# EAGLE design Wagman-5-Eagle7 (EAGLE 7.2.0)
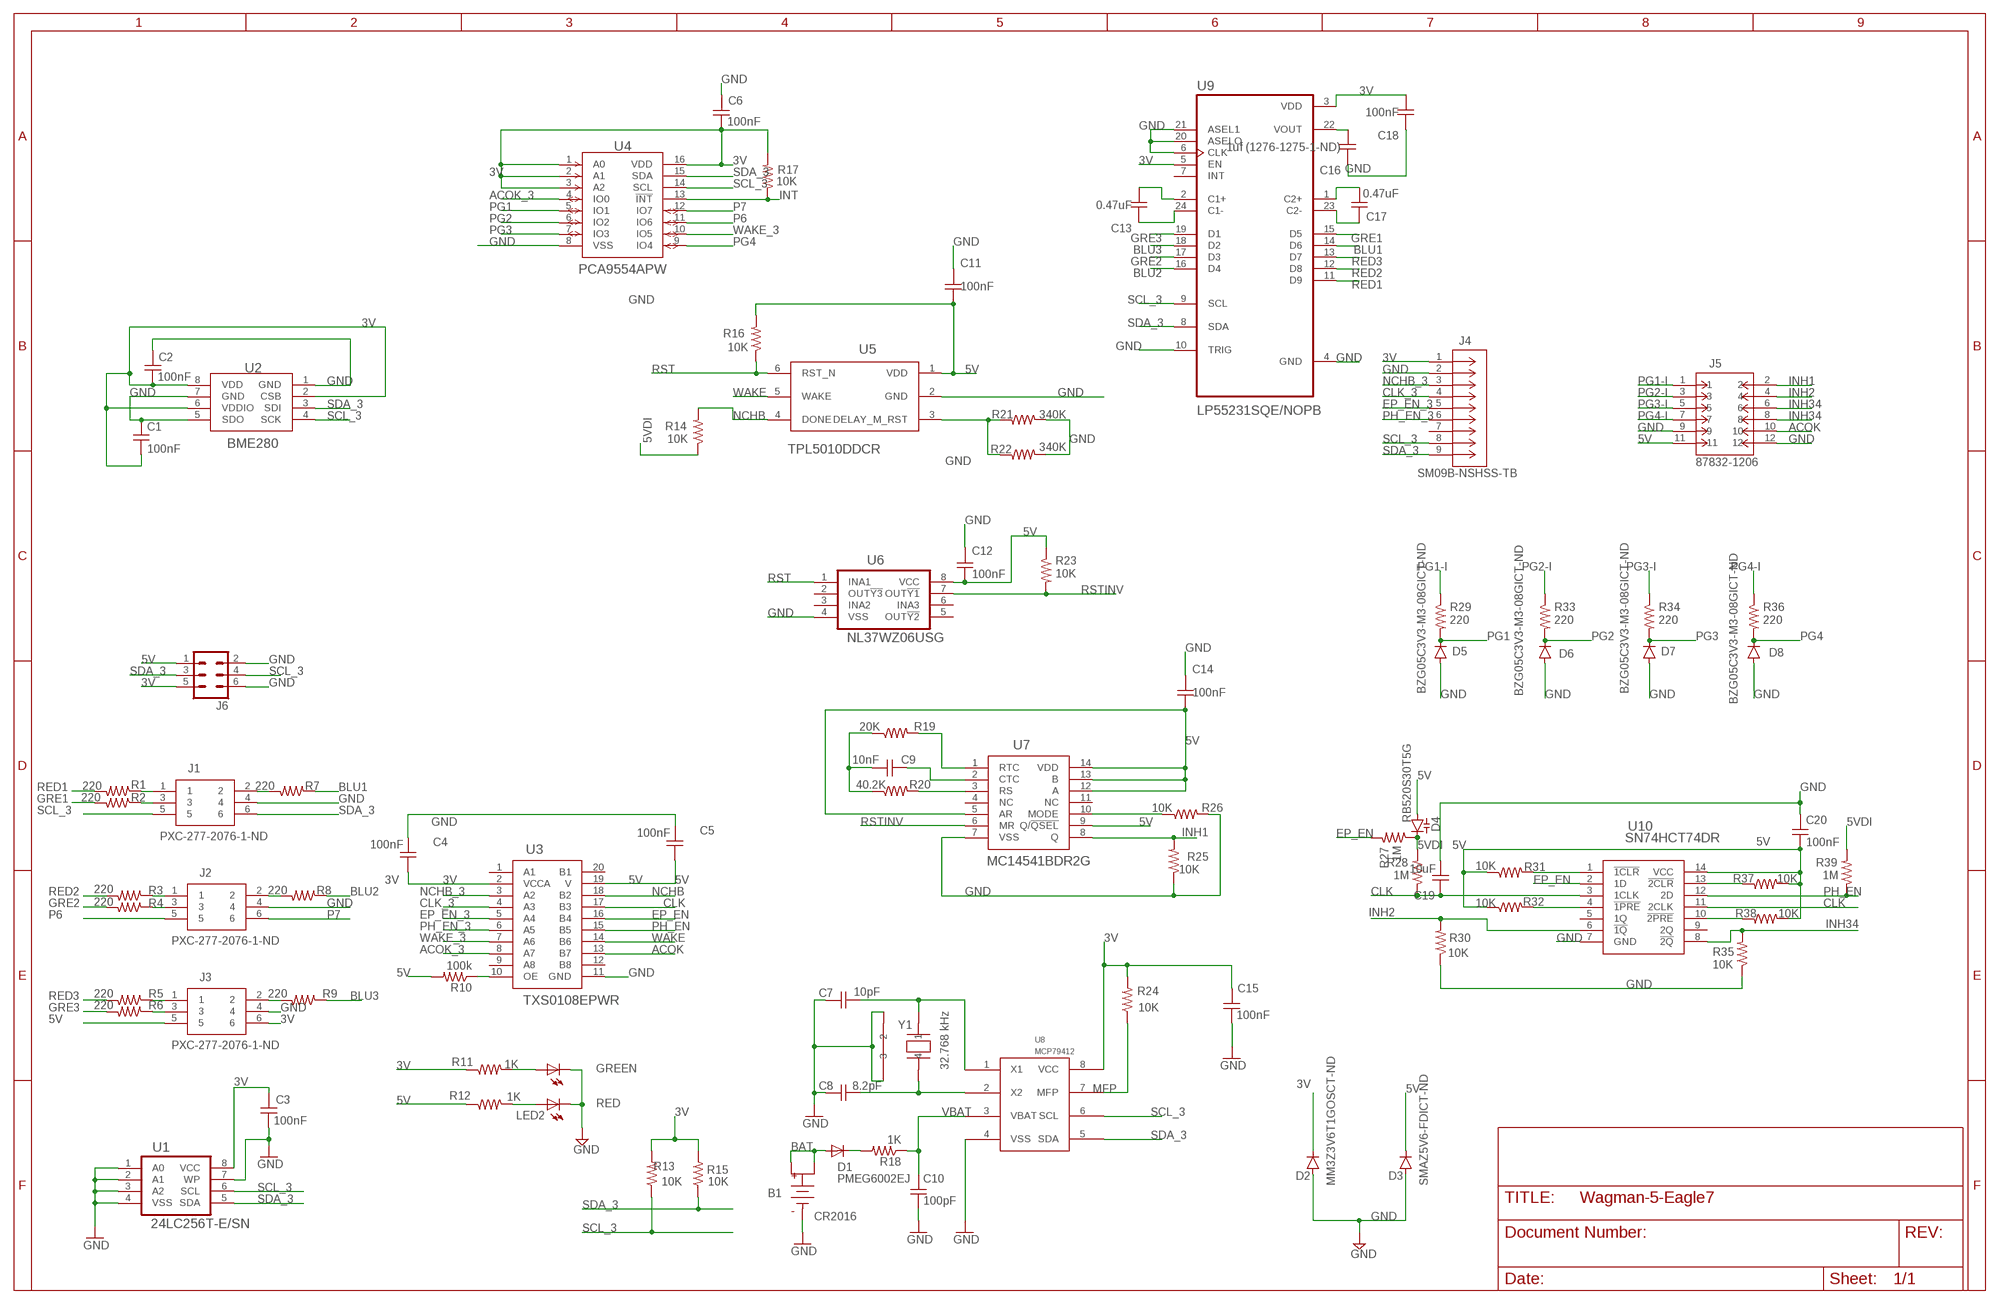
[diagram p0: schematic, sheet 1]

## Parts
B1  CR2016  COIN-CELL-2016-SMT  [BAT-HLD-002-SMT]
C1  100nF  C-USC0805  [C0805]
C2  100nF  C-USC0805  [C0805]
C3  100nF  C-USC0805  [C0805]
C4  100nF  C-USC0805  [C0805]
C5  100nF  C-USC0805  [C0805]
C6  100nF  C-USC0805  [C0805]
C7  10pF  C-USC0805  [C0805]
C8  8.2pF  C-USC0805  [C0805]
C9  10nF  C-USC0805  [C0805]
C10  100pF  C-USC0805  [C0805]
C11  100nF  C-USC0805  [C0805]
C12  100nF  C-USC0805  [C0805]
C13  0.47uF  C-USC0805  [C0805]
C14  100nF  C-USC0805  [C0805]
C15  100nF  C-USC0805  [C0805]
C16  1uf (1276-1275-1-ND)  C-USC0805  [C0805]
C17  0.47uF  C-USC0805  [C0805]
C18  100nF  C-USC0805  [C0805]
C19  10uF  C-USC0805  [C0805]
C20  100nF  C-USC0805  [C0805]
D1  PMEG6002EJ  DIODESOD-323F  [SOD-323F]
D2  MM3Z3V6T1GOSCT-ND  DIODESMA  [SMA-DIODE]
D3  SMAZ5V6-FDICT-ND  DIODESMA  [SMA-DIODE]
D4  RB520S30T5G  BB141  [SOD523]
D5  BZG05C3V3-M3-08GICT-ND  DIODESMA  [SMA-DIODE]
D6  BZG05C3V3-M3-08GICT-ND  DIODESMA  [SMA-DIODE]
D7  BZG05C3V3-M3-08GICT-ND  DIODESMA  [SMA-DIODE]
D8  BZG05C3V3-M3-08GICT-ND  DIODESMA  [SMA-DIODE]
J1  PXC-277-2076-1-ND  [6PIN-PTSM-2.5MM]
J2  PXC-277-2076-1-ND  [6PIN-PTSM-2.5MM]
J3  PXC-277-2076-1-ND  [6PIN-PTSM-2.5MM]
J4  SM09B-NSHSS-TB  [SM09B-NSHSS-TB]
J5  87832-1206  [CON00463_MOL]
J6  MA03-2  [MA03-2]
LED1  GREEN  LEDCHIPLED_0805  [CHIPLED_0805]
LED2  RED  LEDCHIPLED_0805  [CHIPLED_0805]
R1  220  R-US_R0805  [R0805]
R2  220  R-US_R0805  [R0805]
R3  220  R-US_R0805  [R0805]
R4  220  R-US_R0805  [R0805]
R5  220  R-US_R0805  [R0805]
R6  220  R-US_R0805  [R0805]
R7  220  R-US_R0805  [R0805]
R8  220  R-US_R0805  [R0805]
R9  220  R-US_R0805  [R0805]
R10  100k  R-US_R0805  [R0805]
R11  1K  R-US_R0805  [R0805]
R12  1K  R-US_R0805  [R0805]
R13  10K  R-US_R0805  [R0805]
R14  10K  R-US_R0805  [R0805]
R15  10K  R-US_R0805  [R0805]
R16  10K  R-US_R0805  [R0805]
R17  10K  R-US_R0805  [R0805]
R18  1K  R-US_R0805  [R0805]
R19  20K  R-US_R0805  [R0805]
R20  40.2K  R-US_R0805  [R0805]
R21  340K  R-US_R0805  [R0805]
R22  340K  R-US_R0805  [R0805]
R23  10K  R-US_R0805  [R0805]
R24  10K  R-US_R0805  [R0805]
R25  10K  R-US_R0805  [R0805]
R26  10K  R-US_R0805  [R0805]
R27  1M  R-US_R0805  [R0805]
R28  1M  R-US_R0805  [R0805]
R29  220  R-US_R0805  [R0805]
R30  10K  R-US_R0805  [R0805]
R31  10K  R-US_R0805  [R0805]
R32  10K  R-US_R0805  [R0805]
R33  220  R-US_R0805  [R0805]
R34  220  R-US_R0805  [R0805]
R35  10K  R-US_R0805  [R0805]
R36  220  R-US_R0805  [R0805]
R37  10K  R-US_R0805  [R0805]
R38  10K  R-US_R0805  [R0805]
R39  1M  R-US_R0805  [R0805]
U1  24LC256T-E/SN  [SOIC8]
U2  BME280  [8-LGA(2.5X2.5)]
U3  TXS0108EPWR  [PW20]
U4  PCA9554APW  [TSSOP-16]
U5  TPL5010DDCR  TPL5010DDCRDDC0006A_L  [SOT23-6]
U6  NL37WZ06USG  [US-8]
U7  MC14541BDR2G  [SOIC14-3.9MM]
U8  MCP79412  MCP7941X-SOIC-8  [SO08]
U9  LP55231SQE/NOPB  [QFN50P400X400X80-25N]
U10  SN74HCT74DR  [D14]
Y1  32.768 kHz  CRYSTAL-CITIZEN-CM2XXC  [CRYSTAL-CITIZEN-CM2XXC]

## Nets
3V: C1.2 C2.2 C3.1 C4.1 C6.2 C15.1 C18.2 D2.C J3.6 J4.1 J6.5 R11.1 R13.2 R15.2 R17.2 R24.2 U1.8(VCC) U2.2(CSB) U2.6(VDDIO) U2.8(VDD) U3.2(VCCA) U4.1(A0) U4.2(A1) U4.3(A2) U4.16(VDD) U8.8(VCC) U9.3(VDD) U9.5(EN)
5V: C5.1 C11.2 C12.2 C14.2 C20.2 D3.C D4.A J3.5 J5.11 J6.1 R10.2 R12.1 R16.2 R23.1 R31.1 R32.1 R37.2 R38.2 U3.19(V) U5.1(VDD) U6.8(VCC) U7.5(AR) U7.9(Q/!QSEL) U7.12(A) U7.13(B) U7.14(VDD) U10.14(VCC)
5VDI: D4.C R14.1 R27.1 R28.2 R39.2
ACOK: J5.10 U3.13(B7)
ACOK_3: U3.8(A7) U4.4(IO0)
BAT: B1.POS1 B1.POS2 D1.A
BLU1: R7.1 U9.14(D6)
BLU2: R8.1 U9.16(D4)
BLU3: R9.1 U9.18(D2)
CLK: C19.1 R28.1 U3.17(B3) U10.3(1CLK) U10.11(2CLK)
CLK_3: J4.4 U3.4(A3)
EP_EN: R27.2 U3.16(B4) U10.2(1D)
EP_EN_3: J4.5 U3.5(A4)
GND: B1.NEG(B-) C1.1 C2.1 C3.2 C4.2 C5.2 C6.1 C7.2 C8.2 C10.2 C11.1 C12.1 C14.1 C15.2 C16.1 C18.1 C19.2 C20.1 D2.A D3.A D5.A D6.A D7.A D8.A J1.4 J2.4 J3.4 J4.2 J5.9 J5.12 J6.2 J6.6 LED1.C LED2.C R21.2 R22.2 R25.1 R26.2 R30.1 R35.1 U1.1(A0) U1.2(A1) U1.3(A2) U1.4(VSS) U1.7(WP) U2.1(GND) U2.5(SDO) U2.7(GND) U3.11(GND) U4.8(VSS) U5.2(GND) U6.4(VSS) U7.7(VSS) U8.4(VSS) U9.4(GND) U9.6(CLK) U9.10(TRIG) U9.20(ASELO) U9.21(ASEL1) U10.7(GND) Y1.2 Y1.3
GRE1: R2.2 U9.15(D5)
GRE2: R4.2 U9.17(D3)
GRE3: R6.2 U9.19(D1)
INH1: J5.2 R25.2 U7.8(Q)
INH2: J5.4 R30.2 U10.6(!1Q)
INH34: J5.6 J5.8 R35.2 U10.8(!2Q)
INT: R17.1 U4.13(!INT)
MFP: R24.1 U8.7(MFP)
N$1: J1.1 R1.1
N$2: J3.1 R5.1
N$3: J1.3 R2.1
N$4: J1.2 R7.2
N$5: J2.1 R3.1
N$6: R31.2 U10.1(!1CLR)
N$8: J2.2 R8.2
N$10: J3.3 R6.1
N$11: J2.3 R4.1
N$12: J3.2 R9.2
N$13: LED1.A R11.2
N$14: LED2.A R12.2
N$15: C8.1 U8.2(X2) Y1.4
N$17: C7.1 U8.1(X1) Y1.1
N$20: R21.1 R22.1 U5.3(DELAY_M_RST)
N$21: D1.K R18.2
N$24: R10.1 U3.10(OE)
N$28: R32.2 U10.4(!1PRE)
N$30: R38.1 U10.10(!2PRE)
N$33: C17.2 U9.1(C2+)
N$34: C17.1 U9.23(C2-)
N$35: C13.2 U9.2(C1+)
N$36: C13.1 U9.24(C1-)
N$37: C16.2 U9.22(VOUT)
N$45: R37.1 U10.13(!2CLR)
N$84: R20.2 U7.3(RS)
N$85: C9.1 U7.2(CTC)
N$86: R19.2 U7.1(RTC)
N$87: C9.2 R19.1 R20.1
N$88: R26.1 U7.10(MODE)
NCHB: R14.2 U3.18(B2) U5.4(DONE)
NCHB_3: J4.3 U3.3(A2)
P6: J2.5 U4.11(IO6)
P7: J2.6 U4.12(IO7)
PG1: D5.C R29.2 U4.5(IO1)
PG1-I: J5.1 R29.1
PG2: D6.C R33.2 U4.6(IO2)
PG2-I: J5.3 R33.1
PG3: D7.C R34.2 U4.7(IO3)
PG3-I: J5.5 R34.1
PG4: D8.C R36.2 U4.9(IO4)
PG4-I: J5.7 R36.1
PH_EN: R39.1 U3.15(B5) U10.12(2D)
PH_EN_3: J4.6 U3.6(A5)
RED1: R1.2 U9.11(D9)
RED2: R3.2 U9.12(D8)
RED3: R5.2 U9.13(D7)
RST: R16.1 U5.6(RST_N) U6.1(INA1)
RSTINV: R23.2 U6.7(OUT!Y1) U7.6(MR)
SCL_3: J1.5 J4.8 J6.4 R13.1 U1.6(SCL) U2.4(SCK) U4.14(SCL) U8.6(SCL) U9.9(SCL)
SDA_3: J1.6 J4.9 J6.3 R15.1 U1.5(SDA) U2.3(SDI) U4.15(SDA) U8.5(SDA) U9.8(SDA)
VBAT: C10.1 R18.1 U8.3(VBAT)
WAKE: U3.14(B6) U5.5(WAKE)
WAKE_3: U3.7(A6) U4.10(IO5)
Unconnected: J4.7 U3.1(A1) U3.9(A8) U3.12(B8) U3.20(B1) U6.2(OUT!Y3) U6.3(INA2) U6.5(OUT!Y2) U6.6(INA3) U7.4(NC) U7.11(NC) U9.7(INT) U10.5(1Q) U10.9(2Q)

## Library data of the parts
B1 = Wagman-5-e7:COIN-CELL
C1-C20 = Wagman-5-e7:C-US: CAPACITOR, American symbol
D1 = _jc:DIODE
D2 D3 D5-D8 = Wagman:DIODE: Diode
D4 = diode:BB141: Capacity DIODE
J1-J3 = Wagman-5-e7:PXC-277-2076-1-ND
J4 = SM09B-NSHSS-TB(455-2769-1-ND):SM09B-NSHSS-TB
J5 = 0878321210(WM12804-ND):87832-1206; BUILT_BY: EMA_Don; COPYRIGHT: Copyright (C) 2016 Accelerated Designs. All rights reserved; MANUFACTURER_PART_NUMBER: 87832-1206; SOURCELIBRARY: Molex_2018-12-15; VENDOR: Molex Connector Corporation
J6 = con-lstb:MA03-2: PIN HEADER; OC_FARNELL: unknown; OC_NEWARK: unknown
LED1 LED2 = Wagman-4_v1.0:LED: LED
R1-R39 = Wagman-5-e7:R-US_: RESISTOR, American symbol
U1 = Wagman-5-e7:24LC256T-E/SN
U2 = BME280(828-1063-1-ND):BME280
U3 = Wagman-4_v1.0:TXS0108EPWR; MANUFACTURER_PART_NUMBER: TXS0108EPWR; VENDOR: Texas Instruments
U4 = PCA9554APW(568-11905-1-ND):PCA9554APW; BUILT_BY: EMA_UL_Team; MANUFACTURER_PART_NUMBER: PCA9554APW; SOURCELIBRARY: NXP_2011-11-10; VENDOR: NXP
U5 = TPL5010DDC(296-44392-1-ND):TPL5010DDCR; COMPTYPE: IC; MANUFACTURER: Texas Instruments; MOUNTTYPE: SMT; PACKAGEREFERENCE: DDC0006A; PARTNUMBER: TPL5010DDC; PIN_COUNT: 6; REFDES: RefDes; ROHS: Y; TYPE: TYPE; VALUE: Value
U6 = Wagman-5-e7:NL37WZ06USG
U7 = MC14541BDR2G:MC14541BDR2G; MANUFACTURER_PART_NUMBER: SN74HCT74DR; VENDOR: Vendor
U8 = Wagman-5-e7:MCP7941X
U9 = LP55231SQE_NOPB:LP55231SQE/NOPB; DESCRIPTION: 9 channel RGB / White LED driver with internal program memory and integrated charge Pump - WQFN 24-WQFN -30 to 85; DIGI-KEY_PART_NUMBER: 296-39059-1-ND; MF: Texas Instruments; MP: LP55231SQE/NOPB; PACKAGE: WQFN-24 Texas Instruments; PURCHASE-URL: https://pricing.snapeda.com/search/part/LP55231SQE/NOPB/?ref=eda
U10 = SN74HCT74DR:SN74HCT74DR; MANUFACTURER_PART_NUMBER: SN74HCT74DR; VENDOR: Vendor
Y1 = Wagman-5-e7:CRYSTAL-CITIZEN-CM2XXC

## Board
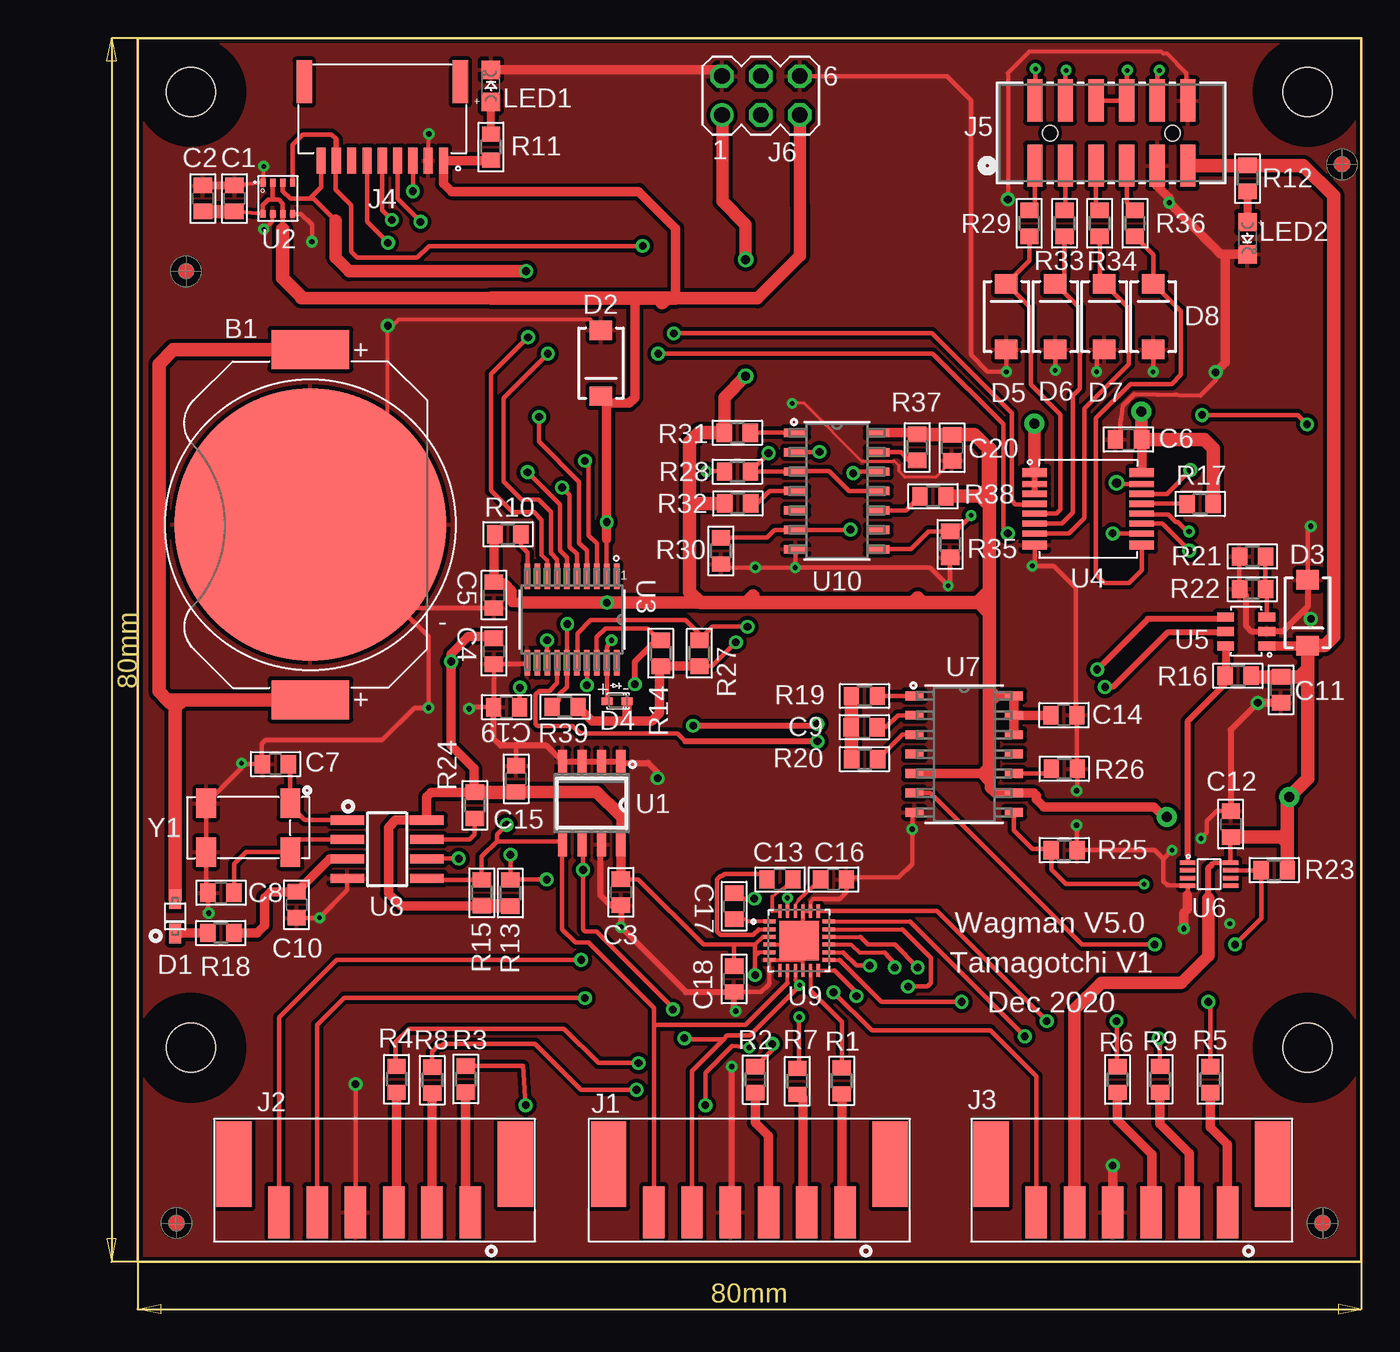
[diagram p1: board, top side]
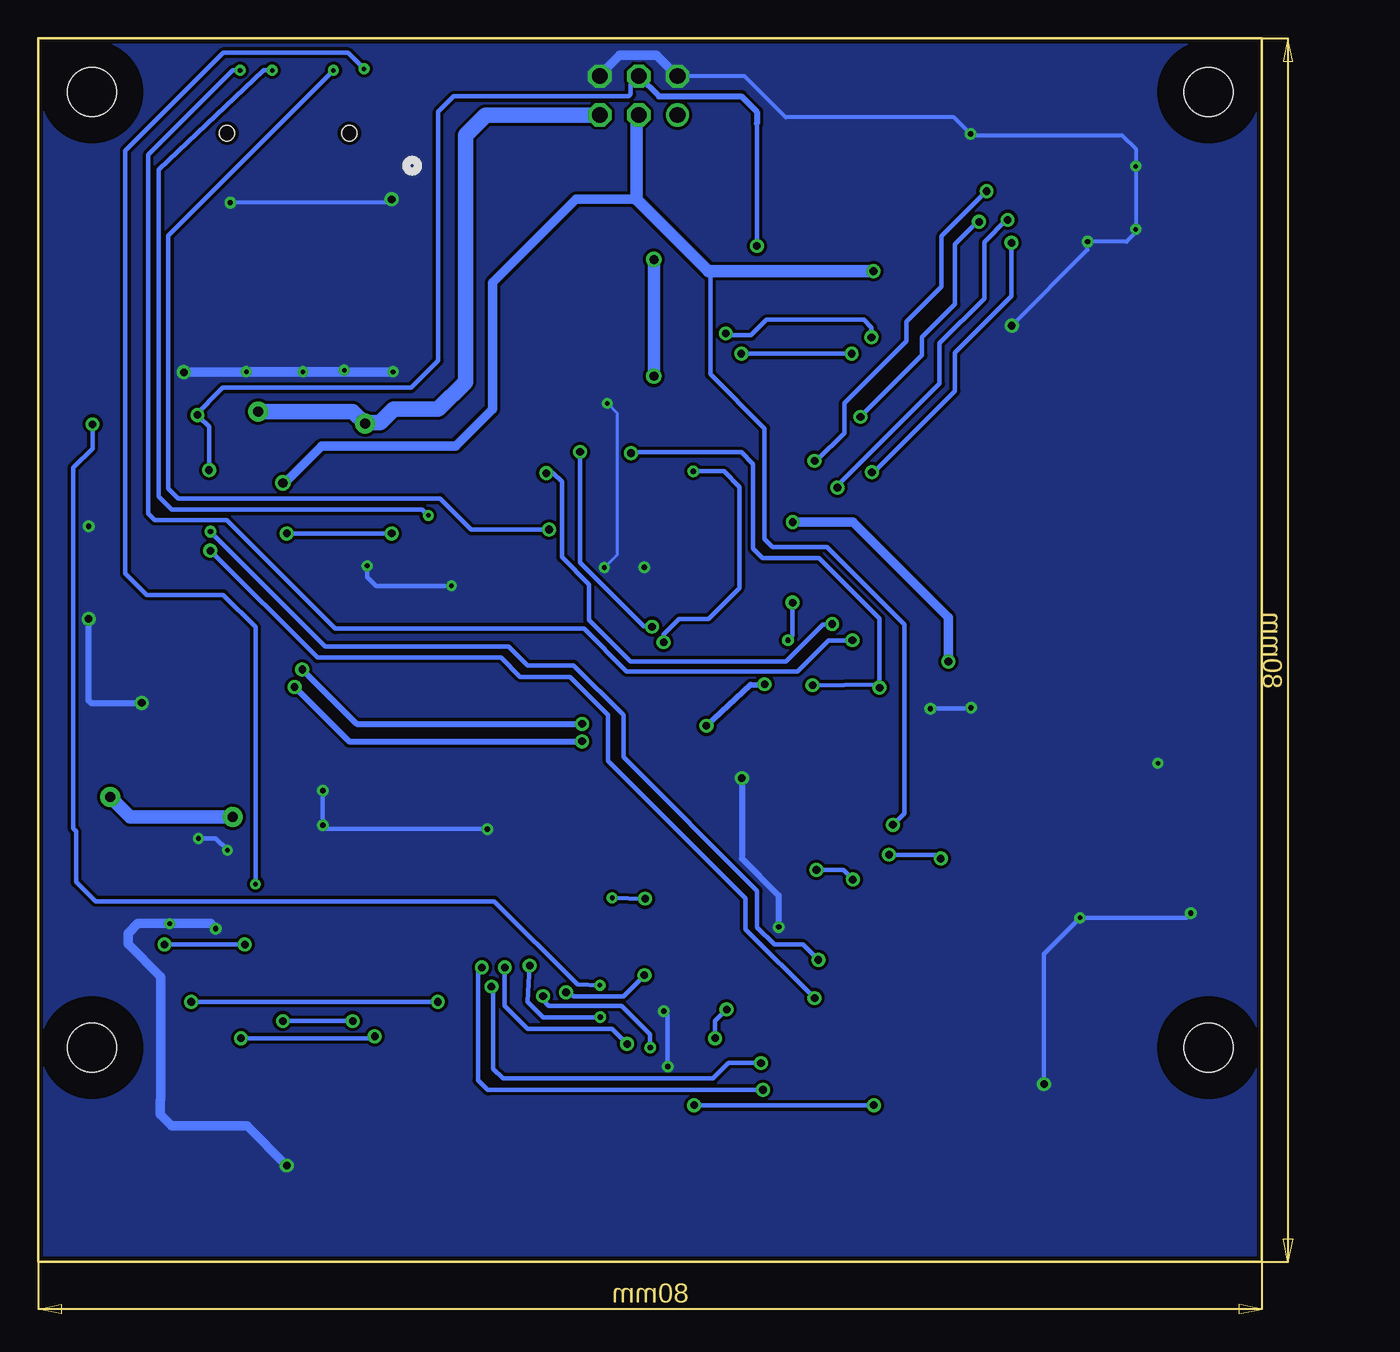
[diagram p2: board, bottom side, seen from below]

Size 82 x 83.38 mm. Coordinates in mm from the lower left corner, seen from the top.
Outline: 2,3.38 82,3.38 82,83.38 2,83.38 2,3.38
Copper layers (1*16): Top 0.035mm / dielectric 1.5mm / Bottom 0.035mm
Design rules "default *": minimum track width 6mil, minimum drill 0.3mm, track to track 0.2mm, track to pad 0.2mm, pad to pad 0.2mm, via to via 0.2mm, smd to smd 6mil, copper to edge 10mil, drill to drill 6mil, minimum pad ring 10mil, minimum via ring 8mil, stop-mask expansion 2mil, vias tented up to drill 0mil, thermal gap 10mil
Holes 3.2 mm at 5.5,17.38 78.5,17.38 78.5,79.88 5.5,79.88
tRestrict: area 2.3,14.2 to 8.7,20.6; area 75.3,14.2 to 81.7,20.6; area 75.3,76.7 to 81.7,83.1; area 2.3,76.7 to 8.7,83.1
bRestrict: area 2.3,14.2 to 8.7,20.6; area 75.3,14.2 to 81.7,20.6; area 75.3,76.7 to 81.7,83.1; area 2.3,76.7 to 8.7,83.1

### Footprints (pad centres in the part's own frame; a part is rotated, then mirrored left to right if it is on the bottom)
BAT-HLD-002-SMT = smd 17.8 x 17.8: NEG 0,0 | smd 2.54 x 5.08: POS1 -11.45,0; POS2 11.45,0
C0805 = smd 1 x 1.2: 1 -0.85,0 | smd 1.006 x 1.2: 2 0.85,0
SOD-323F = smd 1.27 x 0.813: A -1.118,0; K 1.118,0
SMA-DIODE = smd 1.27 x 1.47: A -2.15,0; C 2.15,0
SOD523 = smd 0.7 x 0.5: A 0.7,0; C -0.6,0
6PIN-PTSM-2.5MM = smd 1.4 x 3.4: 1 -6.25,0; 2 -3.75,0; 3 -1.25,0; 4 1.25,0; 5 3.75,0; 6 6.25,0 | smd 2.3 x 5.6: M1 -9.2,-3.15; M2 9.2,-3.15
SM09B-NSHSS-TB = smd 0.6 x 1.7: 1 4,0; 2 3,0; 3 2,0; 4 1,0; 5 0,0; 6 -1,0; 7 -2,0; 8 -3,0; 9 -4,0 | smd 1 x 2.8: 10 5.1,5.15; 11 -5.1,5.15
CON00463_MOL = smd 1 x 2.75: 1 -5,-2.13; 2 -5,2.13; 3 -3,-2.13; 4 -3,2.13; 5 -1,-2.13; 6 -1,2.13; 7 1,-2.13; 8 1,2.13; 9 3,-2.13; 10 3,2.13; 11 5,-2.13; 12 5,2.13 | hole 1: -4,0; 4,0
MA03-2 = drill 1.016: 1 -2.54,-1.27 | drill 1.016 octagon: 2 -2.54,1.27; 3 0,-1.27; 4 0,1.27; 5 2.54,-1.27; 6 2.54,1.27
CHIPLED_0805 = smd 1.2 x 1.2: A 0,-1.05; C 0,1.05
R0805 = smd 1 x 1.2: 1 -0.85,0 | smd 1.006 x 1.2: 2 0.85,0
SOIC8 = smd 0.6 x 1.55: 1 -1.905,-2.7; 2 -0.635,-2.7; 3 0.635,-2.7; 4 1.905,-2.7; 5 1.905,2.7; 6 0.635,2.7; 7 -0.635,2.7; 8 -1.905,2.7
8-LGA(2.5X2.5) = smd 0.35 x 0.5: 1 0.975,-1.025; 2 0.325,-1.025; 3 -0.325,-1.025; 4 -0.975,-1.025; 5 -0.975,1.025; 6 -0.325,1.025; 7 0.325,1.025; 8 0.975,1.025
PW20 = smd 1.676 x 0.356: 1 -2.819,2.925; 2 -2.819,2.275; 3 -2.819,1.625; 4 -2.819,0.975; 5 -2.819,0.325; 6 -2.819,-0.325; 7 -2.819,-0.975; 8 -2.819,-1.625; 9 -2.819,-2.275; 10 -2.819,-2.925; 11 2.819,-2.925; 12 2.819,-2.275; 13 2.819,-1.625; 14 2.819,-0.975; 15 2.819,-0.325; 16 2.819,0.325; 17 2.819,0.975; 18 2.819,1.625; 19 2.819,2.275; 20 2.819,2.925
TSSOP-16 = smd 1.6 x 0.6: 1 -3.5,2.375; 8 -3.5,-2.375; 9 3.5,-2.375; 16 3.5,2.375 | smd 1.6 x 0.4: 2 -3.5,1.625; 3 -3.5,0.975; 4 -3.5,0.325; 5 -3.5,-0.325; 6 -3.5,-0.975; 7 -3.5,-1.625; 10 3.5,-1.625; 11 3.5,-0.975; 12 3.5,-0.325; 13 3.5,0.325; 14 3.5,0.975; 15 3.5,1.625
SOT23-6 = smd 1.1 x 0.6: 1 -1.35,0.95; 2 -1.35,0; 3 -1.35,-0.95; 4 1.35,-0.95; 5 1.35,0; 6 1.35,0.95
US-8 = smd 0.3 x 1: 1 -0.75,-1.4; 2 -0.25,-1.4; 3 0.25,-1.4; 4 0.75,-1.4; 5 0.75,1.4; 6 0.25,1.4; 7 -0.25,1.4; 8 -0.75,1.4
SOIC14-3.9MM = smd 1.2 x 0.58: 1 -3.25,3.81; 2 -3.25,2.54; 3 -3.25,1.27; 4 -3.25,0; 5 -3.25,-1.27; 6 -3.25,-2.54; 7 -3.25,-3.81; 8 3.25,-3.81; 9 3.25,-2.54; 10 3.25,-1.27; 11 3.25,0; 12 3.25,1.27; 13 3.25,2.54; 14 3.25,3.81
SO08 = smd 0.6 x 2.2: 1 -1.905,-2.6; 2 -0.635,-2.6; 3 0.635,-2.6; 4 1.905,-2.6; 5 1.905,2.6; 6 0.635,2.6; 7 -0.635,2.6; 8 -1.905,2.6
QFN50P400X400X80-25N = smd 0.86 x 0.27: 1 -1.935,1.25; 2 -1.935,0.75; 3 -1.935,0.25; 4 -1.935,-0.25; 5 -1.935,-0.75; 6 -1.935,-1.25; 13 1.935,-1.25; 14 1.935,-0.75; 15 1.935,-0.25; 16 1.935,0.25; 17 1.935,0.75; 18 1.935,1.25 | smd 0.27 x 0.86: 7 -1.25,-1.935; 8 -0.75,-1.935; 9 -0.25,-1.935; 10 0.25,-1.935; 11 0.75,-1.935; 12 1.25,-1.935; 19 1.25,1.935; 20 0.75,1.935; 21 0.25,1.935; 22 -0.25,1.935; 23 -0.75,1.935; 24 -1.25,1.935 | smd 2.6 x 2.6: 25 0,0
D14 = smd 1.5 x 0.55: 1 -2.7,3.81; 2 -2.7,2.54; 3 -2.7,1.27; 4 -2.7,0; 5 -2.7,-1.27; 6 -2.7,-2.54; 7 -2.7,-3.81; 8 2.7,-3.81; 9 2.7,-2.54; 10 2.7,-1.27; 11 2.7,0; 12 2.7,1.27; 13 2.7,2.54; 14 2.7,3.81
CRYSTAL-CITIZEN-CM2XXC = smd 1.3 x 1.9: 1 -2.75,-1.6; 2 2.75,-1.6; 3 2.75,1.6; 4 -2.75,1.6

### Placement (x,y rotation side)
B1  13.3,51.58 270 top
C1  8.34,72.9 270 top
C2  6.27,72.9 270 top
C3  33.6,27.55 270 top
C4  25.3,43.3 270 top
C5  25.3,46.98 270 top
C6  66.78,57.15 0 top
C7  11.02,35.93 180 top
C8  7.46,27.51 180 top
C9  49.51,38.34 180 top
C10  12.4,26.73 270 top
C11  76.75,40.78 90 top
C12  73.47,32 270 top
C13  44,28.38 180 top
C14  62.56,39.13 180 top
C15  26.75,34.96 90 top
C16  47.5,28.38 180 top
C17  41,26.63 270 top
C18  41,21.88 90 top
C19  26.12,39.65 180 top
C20  55.25,56.61 90 top
D1  4.46,25.97 270 top
D2  32.3,62.14 270 top
D3  78.5,45.82 270 top
D4  33.4,40.05 180 top
D5  58.8,65.18 90 top
D6  62,65.18 90 top
D7  65.2,65.18 90 top
D8  68.4,65.18 90 top
J1  42,6.63 180 top
J2  17.5,6.63 180 top
J3  67,6.63 180 top
J4  18,75.38 0 top
J5  65.66,77.18 0 top
J6  42.75,79.63 0 top
LED1  25.1,80.26 0 top
LED2  74.56,70.31 180 top
R1  48.05,15.22 90 top
R2  42.39,15.3 90 top
R3  23.46,15.34 90 top
R4  18.93,15.32 90 top
R5  72.13,15.31 90 top
R6  66.06,15.31 90 top
R7  45.14,15.19 270 top
R8  21.27,15.26 270 top
R9  68.84,15.32 270 top
R10  26.21,50.96 180 top
R11  25.11,76.26 90 top
R12  74.56,74.21 270 top
R13  26.38,27.5 270 top
R14  36.2,43.18 90 top
R15  24.5,27.51 270 top
R16  73.94,41.7 0 top
R17  71.47,52.93 0 top
R18  7.45,24.89 180 top
R19  49.52,40.38 0 top
R20  49.53,36.25 0 top
R21  74.89,49.5 180 top
R22  74.89,47.37 180 top
R23  76.31,29 180 top
R24  24.05,33.23 90 top
R25  62.58,30.3 180 top
R26  62.59,35.62 0 top
R27  38.73,43.18 90 top
R28  41.22,55.05 180 top
R29  60.3,71.28 270 top
R30  40.14,49.86 90 top
R31  41.21,57.59 0 top
R32  41.24,52.97 0 top
R33  62.6,71.28 270 top
R34  64.9,71.28 270 top
R35  55.12,50.29 90 top
R36  67.2,71.28 270 top
R37  52.97,56.63 90 top
R38  54,53.44 0 top
R39  29.95,39.66 0 top
U1  31.69,33.38 180 top
U2  11.17,72.91 180 top
U3  30.4,45.38 270 top
U4  64.15,52.62 0 top
U5  74.48,44.6 180 top
U6  72.05,28.73 270 top
U7  56.04,36.58 0 top
U8  18.31,30.36 270 top
U9  45.25,24.38 0 top
U10  47.72,53.78 0 top
U$1  [FIDUCIAL_G10]  5.17,68.15 0 top
U$2  [FIDUCIAL_G10]  80.74,75.13 0 top
U$3  [FIDUCIAL_G10]  4.54,5.92 0 top
U$4  [FIDUCIAL_G10]  79.47,5.92 0 top
Y1  9.24,31.77 180 top

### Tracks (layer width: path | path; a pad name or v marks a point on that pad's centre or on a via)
3V  (via drill 0.5 pad 0.3, 0.5 pad 0.41, 0.65 pad 1.3)
  Top 0.254: U9.5 42.62,23.63 | 42.38,24.13 42.88,24.63 U9.3 | U2.8 C1.2
  Top 0.305: U2.8 10.2,72.47 10.55,72.83 10.8,72.83 | 10.8,72.83 11.25,72.83 11.5,72.58 U2.6 11.49,70.89 | U2.2 10.85,72.88 10.8,72.83 | 8.5,71.88 C1.2 | 72.4,52.95 R17.2 | 27.03,33.88 C15.1 26.75,33.81 | R13.2 26.2,26.64 25.47,26.61 | U3.2 32.67,50.63 32.75,50.63 | C3.1 34.73,28.4 39,24.13 41,24.13 | 41,24.13 C18.2 | 41,24.13 42.38,24.13 42.38,23.38 | 42.62,23.63 42.38,23.38 | 42.38,23.38 v42.38,22.13 | v47.5,21 50,18.5 57.75,18.5 60.75,15.5 J3.6 | U4.3 U4.2
  Top 0.406: 60.62,58.01 60.62,53.6 U4.3
  Top 0.508: 25.08,75.38 R11.1
  Top 0.61: 33.59,28.29 C3.1 U1.8 33.59,32.63 33.5,32.63 | U4.16 67.65,57.13 C6.2 | R15.2 19.22,26.66 18.4,27.48 18.4,31.78 18.89,32.27 U8.8 20.91,33.79 21.2,34.08 R24.2 24,34.13 24,35.63 22.5,37.13 v22.5,42.63 22.5,43.13 23.62,44.26 25.2,44.26 C4.1 | v60.65,58.17 v60.64,58.18 | D2.C 32.5,59.79 | 32.5,59.79 32.8,59.48 32.84,59.51 34.13,59.51 34.51,59.9 34.51,66.38 | 32.5,59.79 32.5,60.13 | 32.5,59.79 arc-90 32.67,59.61 v32.67,51.76 32.67,50.63 | 25.08,75.38 J4.1 22,73.88 22.52,73.36 34.77,73.36 37.18,70.94 37.18,66.38 | 60.62,55.63 60.65,55.61 U4.1 60.62,55.02 60.62,58.01
  Top 0.813: 33.5,32.63 32.02,34.11 C15.1 | 12.7,66.48 12.7,66.38 25.25,66.38 | J6.5 45.29,72.47 45.31,72.45 45.31,69.17 42.52,66.38 37.18,66.38 | v67.63,58.98 C6.2 | v60.64,58.18 60.62,58.16 60.62,58.01 60.62,55.63
  Top 0.889: 12.7,66.48 11.49,67.69 11.49,70.89 | C1.2 C2.2 | R17.2 72.32,56.56 71.73,57.15 C6.2 | R24.2 26.73,34.08 C15.1 | R13.2 R15.2 26.18,26.66 26.2,26.64 | 25.1,66.38 25.25,66.38 34.51,66.38 36.6,66.38 | 36.3,66.08 36.6,66.38 | 37.18,66.38 36.6,66.38
  Bottom 0.305: v42.38,22.13 43.75,20.75 47,20.75 47.25,21 v47.5,21
  Bottom 0.61: v22.5,42.63 22.5,45.51 28.75,51.76 v32.67,51.76
  Bottom 1.016: 51.23,78.36 J6.5 52.75,78.36 54.07,77.04 54.07,60.91 55.85,59.13 58.77,59.13 59.66,58.24 60.58,58.24 v60.64,58.18 | v60.64,58.18 60.58,58.12 | v60.64,58.18 61.44,58.98 v67.63,58.98
5V  (via drill 0.35 pad 0.61, 0.5, 0.6, 0.65 pad 1.3)
  Top 0.3: U6.8 73.45,31.13 C12.2
  Top 0.305: 72.25,29.38 72.35,29.48 U6.8 | D4.A 32.7,42.54 arc90 U3.19 32.68,42.57 32.68,43.61 32.99,43.92 v32.99,44.02
  Top 0.406: 72,27.13 72,29.13 72.25,29.38
  Top 0.61: D3.C 78.88,43.65 78.5,43.65 U5.1 | 57.7,34.74 57.7,35.08 | 57.13,35.31 U7.5 | 57.13,35.31 57.7,35.88 | 57.7,34.74 57.7,34.38 58.04,34.04 U7.9 60.59,34.04 60.75,33.88 60.75,33.63 61.25,33.13 68.43,33.13 69.09,32.47 | 57.7,34.74 57.13,35.31 | U7.13 U7.14 58.21,40.39 | U7.13 U7.12 | 58.21,40.39 57.7,39.88 | 57.7,41.08 57.7,40.9 58.21,40.39 | U10.14 52.86,57.59 R37.2 | U7.13 C14.2 | R10.2 25.3,50.89 C5.1 25.38,47.76 26,47.76 26.5,47.26 26.5,46.48 27.1,46.48 | 32.62,46.48 v32.68,46.48
  Top 0.813: J3.5 63.25,19.88 65,21.63 70.25,21.63 72,23.38 72,27.13 | 27.1,46.48 v32.68,46.48 38.8,46.48 | J6.1 40.23,78.34 40.23,72.72 41.75,71.2 v41.75,68.91 | v41.75,61.29 40.36,59.9 R31.1
  Top 0.889: v77.3,33.78 77.26,33.74 | 57.7,35.08 57.7,35.88 57.7,39.88 57.7,41.08 57.7,45.78 | 57.7,46.48 57.7,45.78 | 57.7,46.48 57.7,47.28 | 57.7,53.58 57.7,52.88 | 57.7,52.88 57.7,47.28 | 38.1,53.38 38.1,56.98 38.71,57.59 R31.1 | 38.1,53.38 38.1,52.56 | 38.1,52.56 38.1,47.18 38.8,46.48 41.8,46.48 | 52.7,46.48 53.3,46.48 | 52.7,46.48 42.3,46.48 | 53.3,46.48 57,46.48 | 41.8,46.48 42.3,46.48 | 57,46.48 57.7,46.48 | 57.7,47.28 57,46.58 57,46.48 | 57.7,45.78 57,46.48 | 42.3,46.48 42.25,46.53 42.25,46.93 41.8,46.48 | 53.3,46.48 53.01,46.77 52.99,46.77 52.7,46.48 | 57.06,53.44 57.56,53.44 57.7,53.58 | 57.7,53.58 57.7,54.08 57.06,53.44 | 57.7,52.88 57.62,52.88 57.06,53.44 | 38.51,52.97 38.1,53.38 | 38.1,52.56 38.51,52.97 | 69.09,32.47 v69.3,32.48 | R32.1 38.51,52.97 | 77.16,30.78 77.16,31.48 | 77.16,30.78 R23.1 | 77.16,31.48 77.16,33.64 v77.3,33.78 | 76.83,31.15 77.16,31.48 | 76.83,31.15 76.83,31.11 77.16,30.78 | R38.2 57.06,53.44 | J5.11 R12.1 78.22,75.06 80.2,73.08 80.2,44.27 79.6,43.67 D3.C 78.5,43.65 78.5,42.18 | R37.2 55.23,57.48 C20.2 56.72,57.46 57.7,56.48 | C12.2 76.83,31.15 | 78.5,42.18 78.5,41.68 | 78.5,41.18 78.5,41.68 | 78.5,41.18 78.5,34.98 v77.3,33.78 | 78,41.63 C11.2 74.86,41.63 R16.2 | 78.05,41.63 78.45,41.63 78.5,41.68 | 78,41.63 78,41.68 78.5,42.18 | 78,41.63 78.05,41.63 | 78.05,41.63 78.5,41.18
  Top 1.016: 57.7,56.48 57.7,54.08
  Bottom 0.305: v32.99,44.02 32.68,44.33 v32.68,46.48
  Bottom 0.813: v41.75,68.91 v41.75,61.29
  Bottom 0.889: v69.3,32.48 76,32.48 v77.3,33.78
5VDI  (via drill 0.35 pad 0.61, 0.5)
  Top 0.305: R28.2 40.35,55.07 v39.19,55.07 | v41.12,43.89 39.55,42.33 R27.1
  Top 0.61: R27.1 R14.1 36.12,42.26 36.12,39.26 35.62,38.76 33.75,38.76 | R39.2 31.7,38.76 33.75,38.76 | 33.75,38.76 34,39.01 D4.C
  Bottom 0.305: v39.19,55.07 37.18,55.07 36.16,54.05 36.16,47.45 38.2,45.42 40.1,45.42 41.12,44.4 v41.12,43.89
ACOK  (via drill 0.3 pad 0.6, 0.5)
  Top 0.305: J5.10 68.66,81.14 v68.8,81.28 | U3.13 v28.77,44.02
  Bottom 0.305: v68.8,81.28 69.3,81.28 74.8,75.78 74.8,52.3 74.39,51.89 69.69,51.89 62.58,44.78 46.32,44.78 43.53,41.99 32.38,41.99 30.35,44.02 v28.77,44.02
ACOK_3  (via drill 0.5)
  Top 0.254: 28.42,49.61 28.77,49.25 U3.8
  Top 0.305: U4.4 60.62,52.91 59.4,52.91 59.15,53.16 59.15,58.88 53.94,64.09 v37.05,64.09 | v27.53,63.83 25.11,61.42 25.11,53.8 26.51,52.4 27.91,52.4 28.42,51.89 28.42,49.61
  Bottom 0.305: v37.05,64.09 37.05,63.96 35.4,63.96 34.38,64.97 28.04,64.97 27.53,64.47 v27.53,63.83
BAT
  Top 0.889: 7.7,63.01 B1.POS1 | 7.7,63.01 6.13,63.01 | 7.7,63.01 4.33,63.01 3.4,62.08 3.4,40.68 3.95,40.13 | 3.95,40.13 6.3,40.13 | 6.3,40.13 B1.POS2 | 4.46,39.62 D1.A | 4.46,39.62 3.95,40.13 | 6.3,40.13 4.97,40.13 4.46,39.62
BLU1  (via drill 0.35 pad 0.61, 0.5 pad 0.3)
  Top 0.254: U9.14 48.12,23.63
  Top 0.305: R7.1 45.25,16.15 v45.25,19.38 | 48.12,23.63 49,22.75 v49.88,22.75
  Bottom 0.305: v45.25,19.38 49,19.38 50,20.38 v49.88,22.75
BLU2  (via drill 0.5 pad 0.3)
  Top 0.254: U9.16 49.25,24.63
  Top 0.305: R8.1 21.25,16.12 21.25,17.13 21.62,17.5 21.88,17.5 22,17.63 28,17.63 31,14.63 v34.62,14.63 | 49.25,24.63 49.75,24.13 51.5,24.13 v53,22.63
  Bottom 0.305: v34.62,14.63 52.62,14.63 53.25,15.25 53.25,22.38 v53,22.63
BLU3  (via drill 0.5 pad 0.3)
  Top 0.254: U9.18 52.5,25.63
  Top 0.305: 52.5,25.63 v60,18.13 | v68.75,18 68.84,17.92 R9.1
  Bottom 0.305: v60,18.13 60.12,18 v68.75,18
CLK  (via drill 0.5, 0.5 pad 0.3)
  Top 0.305: 27,39.62 C19.1 26.98,40.9 v27,40.93 | U3.17 v31.38,41.08 | U10.11 48.5,53.78 47.21,55.07 45.04,55.07 U10.3 R28.1 43.25,56.23 v43.25,56.26
  Bottom 0.305: v31.38,41.08 27.2,41.13 v27,40.93 27,45.45 30.96,49.41 34.66,49.41 35.27,50.01 35.27,55.55 36.04,56.31 43.2,56.31 v43.25,56.26
CLK_3  (via drill 0.5 pad 0.3)
  Top 0.305: U3.4 31.38,49.88 30.88,50.38 30.88,54.38 28.25,57.01 v28.25,58.63 | v20.5,71.38 19,72.88 J4.4
  Bottom 0.305: v28.25,58.63 24.23,62.66 24.23,63.83 22.07,65.99 22.07,69.93 20.61,71.38 v20.5,71.38
EP_EN  (via drill 0.5)
  Top 0.305: U3.16 30.75,42.59 30.75,44.48 31.62,45.34 37.81,45.34 38.73,44.42 R27.2 38.73,44.05 39.59,44.91 v41.88,44.91 | U10.2 45.04,56.34 v46.58,56.34
  Bottom 0.305: v46.58,56.34 46.58,49.1 42.39,44.91 v41.88,44.91
EP_EN_3  (via drill 0.5 pad 0.3)
  Top 0.305: J4.5 18,72.13 v18.62,71.5 | v29.75,54.01 30.25,53.51 30.25,50.13 30.73,49.66 U3.5
  Bottom 0.305: v29.75,54.01 29.75,54.13 23.08,60.8 23.08,63.45 20.16,66.37 20.16,70.05 18.71,71.5 v18.62,71.5
GND  (via drill 0.3 pad 0.6, 0.3 pad 0.61, 0.35, 0.35 pad 0.6, 0.5, 0.5 pad 0.3)
  Top 0.203: C20.1 54.18,54.69 52.16,54.69 51.78,55.07 51.78,55.45 51.53,55.7 49.37,55.7 45.56,59.51 v44.8,59.51 | U1.4 29.79,36.1 32.33,36.1 U1.2 | U1.3 34.21,36.08 34.21,36.01 | 58.83,61.55 58.8,61.55 D5.A | 45.5,23.14 45.5,24.16 arc-90 45.47,24.13 | U9.6 arc-45 43.34,23.14
  Top 0.254: J4.2 v21.05,77.13 | U2.1 10.26,73.99 | v10.26,70.89 10.28,70.89 10.79,71.4 U2.7 | D2.A 31.59,65 19.07,65 18.66,64.59 v18.36,64.59 18.36,56.64 13.5,51.78 | R30.1 40.37,48.78 v45,48.78 42.39,48.78 v42.37,48.8 | 46.2,27.13 46,26.93 U9.20 U9.21 | 43.31,21.69 U9.6 | U9.10 45.5,23.14 43.34,23.14 | U9.4 45.47,24.13 | J5.12 70.58,79.39 70.58,81.1 69.31,82.37 69.06,82.37 68.93,82.5 60.29,82.5 58.9,81.1 v58.9,72.85 | v10.26,75.01 U2.1 | U2.1 C1.1
  Top 0.305: U2.5 12.7,71.88 13.4,71.18 v13.4,70.08 | U10.7 45.02,48.8 v45,48.78 53.8,48.78 v55,47.58 55.12,47.7 R35.1 | C10.2 v13.9,25.88 15.71,27.69 U8.4 | R22.2 R21.2 | 8.53,73.94 C1.1 | v78.7,51.48 78.5,51.28 D3.A | D8.A v68.4,61.58 | D7.A 64.7,62.53 v64.7,61.58 | D6.A v62,61.68 | D5.A v58.8,61.58 | U4.8 60.65,49.03 v60.5,48.88 61.91,48.88 63.34,47.45 63.34,39.2 C14.1 | 46.2,27.13 47.91,27.13 48.35,27.57 C16.1 48.47,28.5 51.75,28.5 52.65,29.4 v52.65,31.68 52.65,32.63 U7.7 | 70.64,27.38 70.65,27.39 U6.4 69.35,27.98 69.06,28.27 69.06,29.73 | 69.06,29.73 68.48,30.3 R25.1 63.4,30.33 v63.4,31.93 | 69.06,29.73 v69.63,30.3 | v71.53,31.07 71.91,31.45 71.91,32.21 72.56,32.85 C12.1 | v63.4,34.18 63.44,34.22 R26.2 63.41,35.65 C14.1 | C14.1 63.5,39.04 | C15.2 26.75,37.13 | v6.65,26.18 6.61,26.18 C8.2 6.49,27.63 Y1.3 Y1.2 8.8,35.68 v8.8,35.98 8.85,35.93 C7.2 10.22,35.88 10.25,35.88 10.12,36.01 10.12,37.26 10.38,37.51 18,37.51 20.1,39.61 v21.02,39.61 21.02,44.26 19.14,46.14 | v16.25,15 J2.4 | v23.68,39.55 23.77,39.65 C19.2 25.3,39.67 C4.2 27.37,42.46 U3.11 | 13.5,51.78 19.14,46.14 | C5.2 23.12,46.13 23.11,46.14 19.14,46.14 | C6.1 66.26,57.48 66.26,58.24 66.31,58.57 66.41,59.36 67.18,60.12 71.47,60.02 72.48,61.04 v72.48,61.55 | 58.83,61.55 58.78,61.6 57.58,61.6 56.48,62.69 56.48,79.33 54.91,80.9 J6.6 | C18.1 arc-45 C18.1 42.77,21.03 43.24,21.51 arc45 43.31,21.69 | 45.5,24.16 U9.21
  Top 0.406: v75.24,39.93 73.47,38.16 C12.1 | R22.2 74.45,46.96 74.45,44.97 74.83,44.6 U5.2 76.88,44.6 78.3,46.02 | D3.A 78.52,47.95 78.52,46.24 78.3,46.02 | v78.71,45.42 78.3,45.83 78.3,46.02 | J1.4 40.85,6.73 v40.85,16.16 | v41.1,19.78 41,19.88 C18.1 37.85,21.03 v33.6,25.28 C3.2 32.93,26.7 32.25,27.38 32.25,30.61 U1.7 | C19.2 25.27,37.66 25.25,37.63 25.75,37.13 26.75,37.13 28.73,37.13 U1.4 U1.3 U1.2 U1.1 33.67,36.01 34.21,36.01 35.38,36.01 36,35.38 v36,35.01
  Top 0.508: C1.1 C2.1 | C11.1 v75.24,39.93
  Top 0.61: J3.4 v65.75,9.68 | 70.64,27.38 70.64,26.43 70.4,26.19 v70.4,25.18 | J6.2 39.8,81.31 LED1.C | J5.9 68.62,75.02 68.62,73.75 69.45,72.93 v69.45,72.63 72.82,69.26 73.12,69.26 | 73.12,69.26 LED2.C | v72.48,61.55 73.12,62.18 73.12,69.26
  Top 0.889: 13.5,51.78 B1.NEG
  Bottom 0.203: v44.8,59.51 44.16,58.88 44.16,49.61 v44.99,48.78 v45,48.78
  Bottom 0.254: J6.2 35.83,80.9 33.14,78.21 22.13,78.21 v21.05,77.13 20.96,77.04 11.14,77.04 10.26,76.15 v10.26,75.01 v10.26,70.89 10.26,70.69 10.87,70.08 v13.4,70.08 13.4,69.55 v18.36,64.59 | v58.9,72.85 59.12,72.63 v69.45,72.63
  Bottom 0.305: v69.63,30.3 70.39,31.07 v71.53,31.07 | v63.4,34.18 v63.4,31.93 63.15,31.68 v52.65,31.68 | v41.1,19.78 40.85,19.53 v40.85,16.16 | v6.65,26.18 6.95,25.88 v13.9,25.88 16.25,23.53 v16.25,15 | v21.02,39.61 21.07,39.55 v23.68,39.55 | v55,47.58 59.91,47.58 60.5,48.16 v60.5,48.88
  Bottom 0.406: v75.24,39.93 75.28,39.89 78.52,39.89 78.71,40.08 v78.71,45.42 | v36,35.01 36,29.75 33.6,27.36 v33.6,25.28
  Bottom 0.61: J6.2 41.56,82.25 44,82.25 45.29,80.96 J6.6 | v58.8,61.58 58.83,61.55 61.94,61.55 | 61.94,61.55 v72.48,61.55 | v68.4,61.58 v64.7,61.58 62.1,61.58 v62,61.68 61.94,61.62 61.94,61.55 | v70.4,25.18 70.72,25.5 v73.41,25.5 75.49,25.5 76.12,24.87 76.12,24.16 73.98,22.02 73.98,14 74.03,13.95 74.03,13.03 73.27,12.27 68.34,12.27 v65.75,9.68
  pour Top (isolate 0.254, rank 6): 2,3.38 82,3.38 82,83.38 2,83.38
  pour Bottom (rank 6, no thermals): 2,3.38 82,3.38 82,83.38 2,83.38
GRE1  (via drill 0.5 pad 0.3)
  Top 0.254: 50.82,23.61 49.2,23.61 48.62,24.13 U9.15
  Top 0.305: R2.2 43.5,17.26 v43.5,17.63 | 50.82,23.61 51.5,22.88 v51.5,22.63
  Bottom 0.305: v43.5,17.63 44.5,18.63 50,18.63 51.5,20.13 v51.5,22.63
GRE2  (via drill 0.5 pad 0.3)
  Top 0.254: U9.17 52,25.13
  Top 0.305: R4.2 18.88,16.23 18.88,17.75 19.75,18.63 29.88,18.63 32.12,16.38 v34.75,16.38 | 52,25.13 53.88,23.25 53.88,21.63 53.62,21.38 v52.38,21.38
  Bottom 0.305: v34.75,16.38 36.88,16.38 37.88,15.38 51.62,15.38 52.25,16 52.25,21.25 v52.38,21.38
GRE3  (via drill 0.5)
  Top 0.254: 47.03,26.31 47.03,26.32
  Top 0.305: R6.2 66.01,16.22 v66.01,19.13 | v61.44,19.13 54.25,26.32 47.03,26.32 | 47.03,26.31 U9.19
  Bottom 0.305: v66.01,19.13 v61.44,19.13
INH1  (via drill 0.3 pad 0.6)
  Top 0.305: J5.2 60.7,79.35 v60.7,81.38 | v67.8,28.08 62.7,28.08 61.73,29.05 R25.2 61.65,30.38 60.5,30.38 59.29,31.59 U7.8
  Bottom 0.305: v67.8,28.08 67.8,44.88 69.9,46.98 74.9,46.98 76.3,48.38 76.3,76.03 69.9,82.43 61.75,82.43 v60.7,81.38
INH2  (via drill 0.3 pad 0.6, 0.5 pad 0.41)
  Top 0.305: J5.4 62.66,81.24 v62.7,81.28 | 40.16,50.69 R30.2 40.18,50.75 43.15,50.75 43.64,51.24 U10.6 48.59,51.24 v48.61,51.26
  Bottom 0.305: 62.6,81.38 v62.7,81.28 73.5,70.48 73.5,53.93 72.87,53.29 55.72,53.29 53.69,51.26 v48.61,51.26
INH34  (via drill 0.3 pad 0.6)
  Top 0.305: J5.6 J5.8 66.66,81.34 v66.7,81.28 | v56.5,52.18 55.46,51.14 R35.2 53.7,51.14 52.55,49.99 50.44,49.99 U10.8
  Bottom 0.305: v56.5,52.18 56.9,52.58 73.29,52.58 74.14,53.43 74.14,74.79 67.27,81.28 v66.7,81.28
INT
  Top 0.305: U4.13 70.61,52.95 R17.1
MFP
  Top 0.305: U8.7 23.71,30.99 24.05,31.33 R24.1
N$1
  Top 0.61: J1.1 48.05,6.83 R1.1
N$2
  Top 0.61: R5.1 72.13,12.18 73.25,11.06 J3.1
N$3
  Top 0.61: J1.3 43.39,6.77 43.25,6.91 43.25,11.63 42.39,12.49 R2.1
N$4
  Top 0.61: J1.2 45.5,6.88 45.5,14.13 45.29,14.34 R7.2
N$5
  Top 0.61: J2.1 23.46,6.92 R3.1
N$6
  Top 0.305: U10.1 R31.2
N$8
  Top 0.61: J2.2 21.27,6.64 R8.2
N$10
  Top 0.61: J3.3 68.29,6.67 68.29,10.43 66.06,12.66 R6.1
N$11
  Top 0.61: J2.3 18.93,6.81 R4.1
N$12
  Top 0.61: J3.2 70.77,6.65 70.77,10.49 68.84,12.43 R9.2
N$13
  Top 0.508: R11.2 LED1.A
N$14
  Top 0.508: R12.2 LED2.A
N$15
  Top 0.305: U8.2 12.62,30.99 11.99,30.37 Y1.4 9.09,30.17 8.31,29.39 C8.1
N$17
  Top 0.305: 11.99,33.19 Y1.1 | Y1.1 11.99,33.19 | U8.1 12.91,32.27 11.99,33.19 | Y1.1 11.99,35.81 C7.1
N$20
  Top 0.305: R21.1 R22.1 75.83,47.36 U5.3
N$21
  Top 0.61: R18.2 4.5,24.89 D1.K
N$24
  Top 0.305: U3.10 27.5,48.22 27.5,49.76 27.07,50.19 R10.1
N$28
  Top 0.305: U10.4 43.3,53.78 42.49,52.97 R32.2
N$30
  Top 0.305: U10.10 52.22,52.51 R38.1
N$33
  Top 0.254: U9.1 | U9.1 41.9,25.63 41.75,25.78 C17.2
  Top 0.305: 41.1,25.63 C17.2
N$34  (via drill 0.3 pad 0.25, 0.5 pad 0.3)
  Top 0.305: U9.23 44.5,26.89 v44.48,27.18 | v42.32,27.13 41.1,27.13 C17.1
  Bottom 0.305: v44.48,27.18 v42.32,27.13
N$35
  Top 0.254: 42.62,25.13 U9.2
  Top 0.305: 42.62,25.13 42.25,24.75 40.12,24.75 39.88,25 39.88,28.38 40.12,28.63 40.25,28.63 40.38,28.75 42.75,28.75 43.12,28.38 C13.2
N$36
  Top 0.203: 43.5,27.26 43.91,27.59 44.48,28.02
  Top 0.254: U9.24 43.5,26.32 43.5,27.26
  Top 0.305: 44.48,28.02 C13.1
N$37
  Top 0.203: U9.22 45.03,26.75 45.23,27.08
  Top 0.254: 45.23,27.08 C16.2
  Top 0.305: 46.77,28.27 C16.2
N$45
  Top 0.305: U10.13 51.9,56.32 52.44,55.78 R37.1
N$84
  Top 0.305: R20.2 50.56,36.42 51.99,37.85 U7.3
N$85
  Top 0.305: U7.2 51.7,39.12 50.92,38.34 C9.1
N$86
  Top 0.305: R19.2 50.48,40.39 U7.1
N$87
  Top 0.889: R19.1 C9.2 48.68,38.34 R20.1
N$88
  Top 0.305: U7.10 61.43,35.31 R26.1
NCHB  (via drill 0.5)
  Top 0.305: U3.18 32.02,44.22 32.58,44.78 35.33,44.78 36.08,44.03 R14.2
  Top 0.406: U5.4 73,45.42 68.04,45.42 v64.74,42.12 | v46.45,38.56 46.32,38.43 v38.32,38.43 | v34.51,41.15 34.51,42.62 35.92,44.03 R14.2
  Bottom 0.406: v64.74,42.12 61.18,38.56 v46.45,38.56 | v38.32,38.43 35.43,41.1 v34.51,41.15
NCHB_3  (via drill 0.5 pad 0.3)
  Top 0.305: J4.3 v20,73.38 | v31.25,55.76 31.5,55.51 31.5,50.88 32.02,50.36 U3.3
  Bottom 0.305: v31.25,55.76 31.12,55.76 29.3,57.58 29.3,59.51 25.24,63.58 25.24,64.85 22.95,67.13 22.95,70.44 v20.01,73.38 v20,73.38
P6  (via drill 0.5 pad 0.3)
  Top 0.305: J2.5 13.75,18.88 15.5,20.63 v31.25,20.63 | v70.75,49.88 68.98,51.65 U4.11
  Bottom 0.305: v70.75,49.88 63.75,42.88 51.75,42.88 50.5,41.63 47.25,41.63 44.75,39.13 44.75,36.13 35.75,27.13 35.75,25.13 v31.25,20.63
P7  (via drill 0.35 pad 0.61, 0.5 pad 0.3)
  Top 0.305: J2.6 11.25,19.38 15,23.13 v31,23.13 | U4.12 67.69,52.26 69.38,52.26 69.88,51.76 70,51.76 70.62,51.13 v70.75,51.13
  Bottom 0.305: v70.75,51.13 63.25,43.63 51.25,43.63 50,42.38 47,42.38 43.75,39.13 43.75,36.38 35,27.63 35,25.25 33.88,24.13 32,24.13 v31,23.13
PG1
  Top 0.305: 60.4,70.33 R29.2 60.3,68.83 D5.C 60.4,65.73 60.4,60.73 62.34,58.78 62.34,52.58 62.06,52.3 U4.5
PG1-I
  Top 0.305: J5.1 60.66,72.49 R29.1
PG2
  Top 0.305: 63,70.03 R33.2 62.6,67.93 D6.C 63.6,65.73 63.6,60.48 63.15,60.03 63.15,52.38 62.41,51.65 U4.6
PG2-I
  Top 0.305: J5.3 62.66,72.19 R33.1
PG3
  Top 0.305: U4.7 62.9,51 63.91,52 63.91,59.18 66.8,62.07 66.8,65.73 D7.C 64.9,67.63 R34.2
PG3-I
  Top 0.305: J5.5 64.66,72.37 R34.1
PG4
  Top 0.305: U4.9 67.65,48.63 66.8,47.78 65.2,47.78 64.65,48.33 64.65,58.54 66.9,60.78 69.6,60.78 70.2,61.38 70.2,65.53 D8.C 68.4,69.23 R36.2
PG4-I
  Top 0.305: J5.7 66.66,72.67 R36.1
PH_EN  (via drill 0.5)
  Top 0.305: R39.1 29.56,40.13 29.56,40.46 30.07,40.98 U3.15 30.09,42.58 v30.09,45.09 | v48.79,54.94 48.9,55.05 U10.12
  Bottom 0.305: v48.79,54.94 48.33,54.94 47.77,54.38 47.77,49.46 45.99,47.68 45.99,45.34 43.27,42.62 33.11,42.62 30.7,45.04 30.14,45.04 v30.09,45.09
PH_EN_3  (via drill 0.5 pad 0.3)
  Top 0.305: J4.6 17,71.38 v18.38,70 | U3.6 30.07,49.43 29.62,49.88 29.62,52.88 v27.49,55.01
  Bottom 0.305: v27.49,55.01 27.37,55.01 22.07,60.31 22.07,62.82 18.38,66.51 v18.38,70
RED1
  Top 0.254: U9.11 46,21.13
  Top 0.305: 46,21.13 48.05,19.09 R1.2
RED2  (via drill 0.35 pad 0.61, 0.5 pad 0.3)
  Top 0.254: U9.12 47.56,22.45
  Top 0.305: v42,17.4 40.88,17.5 39.12,15.75 v39.12,13.63 | v27.38,13.63 27.19,16.19 R3.2 | v49,20.75 49,21 47.56,22.45
  Bottom 0.305: v42,17.4 42,18.25 43.88,20.13 48.62,20.13 49,20.5 v49,20.75 | v39.12,13.63 v27.38,13.63
RED3  (via drill 0.5 pad 0.3)
  Top 0.254: U9.13 47.88,23.13
  Top 0.305: 47.88,23.13 50.62,20.38 v55.88,20.38 | v72,20.38 72.13,20.25 R5.2
  Bottom 0.305: v55.88,20.38 v72,20.38
RST
  Top 0.254: 70.63,30 70.65,29.98
  Top 0.305: 73.09,41.17 R16.1 | U6.1 70.65,29.98
  Top 0.406: 73.09,41.17 70.63,38.71 70.63,30
  Top 0.508: U5.6 73.13,41.76 R16.1
RSTINV  (via drill 0.5 pad 0.3)
  Top 0.3: U6.7 75.44,28.98 R23.2
  Top 0.305: U7.6 53.84,34.04 63.75,24.13 v68.5,24.13 | v73.75,24.13 75.46,25.84 R23.2
  Bottom 0.305: v68.5,24.13 v73.75,24.13
SCL_3  (via drill 0.3 pad 0.55, 0.5 pad 0.3, 0.5 pad 0.41)
  Top 0.254: U9.9 45,21.79 v45.28,21.46
  Top 0.305: 15,76.78 14.7,77.08 12.8,77.08 12.14,76.42 U2.4 | J4.8 15,76.78 | 40.31,17.94 40.55,18.21 42.05,18.21 45.28,21.41 v45.28,21.46 | 40.31,17.94 38.25,15.88 J1.5 | U8.6 20.94,29.75 v23,29.75 | v26.38,30 R13.1 26.41,28.38 v28.75,28.38 | v31.12,29 31.12,30.68 U1.6 31.12,30.61 31.12,25.13 31.25,25 32,25 37,20 v37,19.88 | v37.75,18 37.81,17.94 40.31,17.94 | 15,76.78 14.95,76.73 14.95,73.48 15.97,72.47 15.97,69.42 16.35,69.04 20.29,69.04 21.05,69.8 v35.02,69.8 | v78.45,58.14 77.84,58.75 v71.6,58.75 | v70.83,55.15 69.28,53.6 U4.14
  Bottom 0.305: v23,29.75 23.25,30 v26.38,30 | v28.75,28.38 29.38,29 v31.12,29 | v37,19.88 37.75,19.13 v37.75,18 | v35.02,69.8 35.02,77.8 35.02,78.31 | v45.28,21.46 46.76,21.52 52.19,26.95 78.25,26.95 79.52,28.22 79.52,31.52 79.72,31.73 79.72,55.3 78.45,56.57 v78.45,58.14 | v71.6,58.75 71.47,58.62 | v70.83,55.15 70.83,57.99 71.47,58.62 | 71.47,58.62 71.85,58.62 69.94,60.53 57.63,60.53 55.85,62.31 55.85,78.56 54.83,79.58 43.4,79.58 43.27,79.71 43.27,80.34 42.75,80.87 J6.4
  Bottom 0.406: J6.4 41.43,79.58 36.04,79.58 35.02,78.56 35.02,77.8
SDA_3  (via drill 0.5, 0.5 pad 0.41, 0.6)
  Top 0.254: 44.5,21.63 U9.8
  Top 0.305: U2.3 11.5,73.38 12,72.88 13.25,72.88 | 13.25,72.88 14,73.63 J4.9 | 44.5,21.63 41.75,18.88 35.75,18.88 | 35.75,18.88 35.75,20 31.5,24.25 30.62,24.25 29.75,25.13 29.75,30.64 U1.5 29.59,30.88 25.5,30.88 | 35.75,18.88 J1.6 | U8.5 20.91,28.36 R15.1 24.5,29.88 25.5,30.88 | 14.95,71.45 13.53,72.88 13.25,72.88 | v66.01,54.31 66.07,54.25 U4.15 | 25.5,30.88 25.5,31.32 v26.13,31.95
  Top 0.813: v27.4,68.15 15.84,68.15 14.95,69.04 14.95,71.45
  Bottom 0.305: v26.13,31.95 25.37,32.72 25.37,45.04 30.45,50.12 34,50.12 34.51,50.62 34.51,57.86 38.07,61.42 38.07,68.15
  Bottom 0.61: 42.89,72.85 46.83,72.85 52.29,67.39 52.29,59.13 54.7,56.72 63.47,56.72 65.88,54.31 v66.01,54.31
  Bottom 0.813: 42.77,78.31 42.89,78.18 42.89,72.85 38.2,68.15 38.07,68.15 v27.4,68.15
  Bottom 1.016: J6.3 42.77,78.34 42.77,78.31
VBAT
  Top 0.61: U8.3 14.54,29.72 C10.1 10.7,27.58 10.3,27.18 10.3,25.38 9.81,24.89 R18.1
WAKE  (via drill 0.5)
  Top 0.305: U3.14 29.43,42.55 29.43,41.23 28.92,40.72 28.29,40.72 28.04,40.46 28.04,38.56 28.16,38.43 30.45,38.43 30.96,37.92 37.31,37.92 37.81,37.42
  Top 0.406: U5.5 73.06,44.53 69.31,44.53 65.75,40.97 v65.25,40.97 | v46.45,37.42 37.81,37.42
  Bottom 0.406: v65.25,40.97 61.69,37.42 v46.45,37.42
WAKE_3  (via drill 0.5)
  Top 0.305: U4.10 v65.75,51.01 | v58.9,51.01 58.59,51.31 58.59,58.14 53.97,62.77 v36.04,62.77 | v28.82,62.77 25.93,59.87 25.93,54.38 27.09,53.22 28.21,53.22 29.03,52.4 29.03,49.71 29.43,49.31 U3.7
  Bottom 0.305: v65.75,51.01 v58.9,51.01 | v36.04,62.77 v28.82,62.77

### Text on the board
tPlace: + | -
tNames: Wagman V5.0 | Tamagotchi V1 | Dec 2020

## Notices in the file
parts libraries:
dicons: Copyright (C) 2004, Bob Starr (rtzaudio@mindspring.com)
